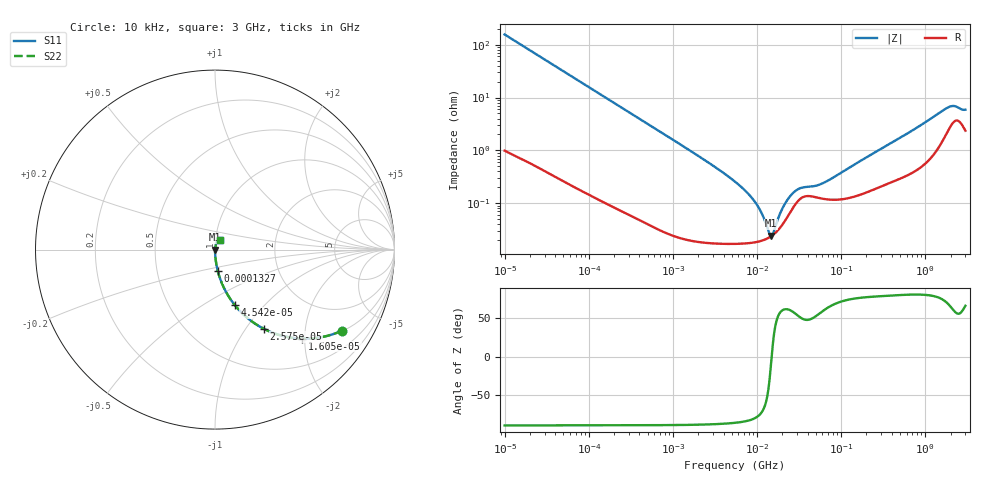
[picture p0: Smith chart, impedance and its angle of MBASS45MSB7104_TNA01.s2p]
! MBASS45MSB7104_TNA01  S-PARAMETER MODEL  ( Standard Model )
! Model Generated by TAIYO YUDEN Corporation (http://www.ty-top.com)
! Version 1.0
! TAIYO YUDEN Control No. 220601
! Copyright(c) 2013 TAIYO YUDEN CO.,LTD. All Rights Reserved.
! Product Description (link to TY-COMPAS)
! https://ds.yuden.co.jp/TYCOMPAS/or/detail?pn=MBASS45MSB7104KTNA01&u=M
! Products Name : Multilayer Ceramic Capacitors
! Characteristics :
!  Capacitance : 0.1 [uF] , Rated Voltage : 630 [V] , TCC : X7R
!  Case Size : 4.5 x 3.2 / 0.177 x 0.126 [mm/inch] , Thickness : 2.5 / 0.098 [mm/inch]
!  (Conditions: Temperature = 25 [degC] , DC Bias Voltage = 0 [V])
! External Node Assignments :
!  1  o---| |---o  2
! GND o---------o GND
! Frequency Range : 10kHz  -  3GHz  [ 401 STEP ]
# MHZ S RI R 50
! Freq[MHz].  S11 Real  S11 Imag  S21 Real  S21 Imag  S12 Real  S12 Imag  S22 Real  S22 Imag
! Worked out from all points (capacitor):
!   401 points, 10 kHz to 3 GHz, reference 50 ohm
!   read as one part in series: C = 102 nF near 10.65 kHz
!   lowest |Z| = 24.2 mohm at 14.56 MHz (marker M1)
!   series resonance near 14.94 MHz, so ESL is about 1.1 nH
!   S11 on the Smith chart (normalised r, x): 10 kHz: 1.02, -3.12; 16.05 kHz: 1.01, -1.95; 25.75 kHz: 1.01, -1.22; 45.42 kHz: 1.01, -0.69; 132.7 kHz: 1.00, -0.24; 3 GHz: 1.05, +0.11
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0.01  0.708 -0.4515  0.292 0.4515  0.292 0.4515  0.708 -0.4515
0.016047  0.4874 -0.4964  0.5126 0.4964  0.5126 0.4964  0.4874 -0.4964
0.02575  0.272 -0.4412  0.728 0.4412  0.728 0.4412  0.272 -0.4412
0.045421  0.109 -0.3076  0.891 0.3076  0.891 0.3076  0.109 -0.3076
0.082683  0.0366 -0.1834  0.9634 0.1834  0.9634 0.1834  0.0366 -0.1834
0.132681  0.0151 -0.1172  0.9849 0.1172  0.9849 0.1172  0.0151 -0.1172
0.683653  0.000856 -0.0233  0.9991 0.0233  0.9991 0.0233  0.000856 -0.0233
5.477226  0.000176 -0.00256  0.9998 0.00256  0.9998 0.00256  0.000176 -0.00256
9.6612  0.000184 -0.000993  0.9998 0.000993  0.9998 0.000993  0.000184 -0.000993
11.31085  0.000195 -0.000629  0.9998 0.000629  0.9998 0.000629  0.000195 -0.000629
13.66633  0.000221 -0.000202  0.9998 0.000202  0.9998 0.000202  0.000221 -0.000202
14.55585  0.000234 -5.97e-05  0.9998 5.97e-05  0.9998 5.97e-05  0.000234 -5.97e-05
15.50326  0.000252 8.42e-05  0.9997 -8.42e-05  0.9997 -8.42e-05  0.000252 8.42e-05
20.5901  0.000418 0.000757  0.9996 -0.000757  0.9996 -0.000757  0.000418 0.000757
25.67485  0.000735 0.00125  0.9993 -0.00125  0.9993 -0.00125  0.000735 0.00125
32.0153  0.00118 0.00149  0.9988 -0.00149  0.9988 -0.00149  0.00118 0.00149
45.28751  0.00134 0.00158  0.9987 -0.00158  0.9987 -0.00158  0.00134 0.00158
70.41703  0.00118 0.00243  0.9988 -0.00243  0.9988 -0.00243  0.00118 0.00243
374.4521  0.00256 0.0129  0.9974 -0.0129  0.9974 -0.0129  0.00256 0.0129
1869.516  0.0265 0.0577  0.9735 -0.0577  0.9735 -0.0577  0.0265 0.0577
2188.735  0.0367 0.0558  0.9633 -0.0558  0.9633 -0.0558  0.0367 0.0558
3000  0.0258 0.0513  0.9742 -0.0513  0.9742 -0.0513  0.0258 0.0513
